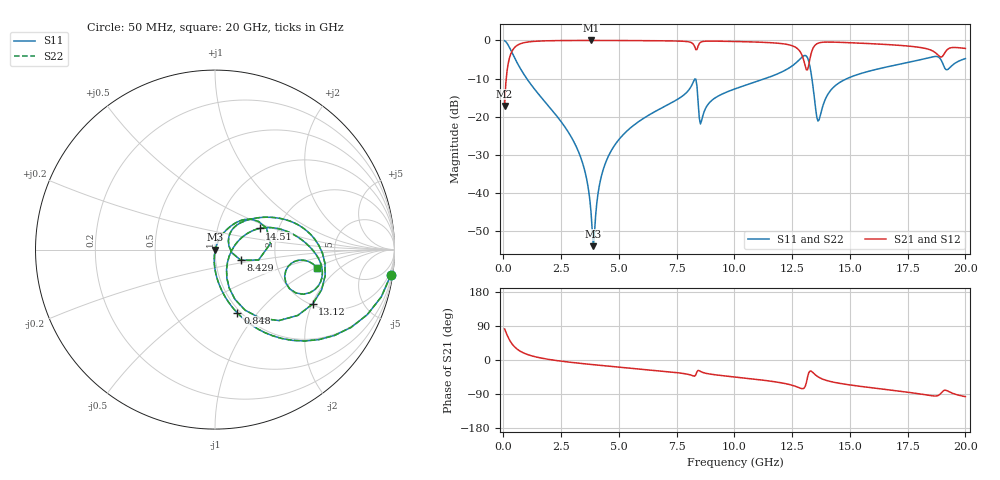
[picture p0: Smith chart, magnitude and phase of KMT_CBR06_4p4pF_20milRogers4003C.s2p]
! Data measured by Modelithics Inc. support@modelithics.com 813-866-6335
! KEMET CBR0603 4.4pF, Pad Width= 0.851mm, Pad Length= 0.64mm, Pad Gap= 0.62mm, 20mil Rogers 4003C substrate Data, January 2022
# hz S ma R 50
! 2 Port Network Data from SP1.SP block
! freq  magS11  angS11  magS21  angS21  magS12  angS12  magS22  angS22
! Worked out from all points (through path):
!   401 points, 50 MHz to 20 GHz, reference 50 ohm
!   highest |S21| = -0.02 dB at 3.791 GHz (marker M1); lowest = -17.2 dB at 50 MHz (marker M2)
!   group delay of S21, straight-line fit = 15.7 ps
!   lowest |S11| = -54.0 dB at 3.89 GHz (marker M3), VSWR 1.00, Z = 50.2 - j0.0729 ohm
!   |S11| at or under -10 dB: 1.007 GHz to 11.34 GHz (10.34 GHz wide, 167 % of centre); 13.35 GHz to 14.88 GHz (1.526 GHz wide, 10.8 % of centre)
!   |S22| runs from -54.0 to -0.1 dB; largest |S21 - S12| = 0
!   S11 on the Smith chart (normalised r, x): 50 MHz: 1, -14; 848 MHz: 0.97, -0.79; 8.429 GHz: 1.33, -0.16; 13.12 GHz: 2.04, -2.02; 14.51 GHz: 1.60, +0.41; 20 GHz: 3.40, -1.02
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5e7  0.9904 -8.1  0.138 81.9  0.138 81.9  0.9904 -8.1
2.99375e8  0.7657 -40.9  0.6424 49.0  0.6424 49.0  0.7657 -40.9
8.48e8  0.3742 -70.6  0.9263 19.3  0.9263 19.3  0.3742 -70.6
3.391625e9  0.02657 -95.3  0.9977 -9.3  0.9977 -9.3  0.02657 -95.3
3.641e9  0.01314 -92.5  0.9979 -10.8  0.9979 -10.8  0.01314 -92.5
3.790625e9  0.005649 -81.5  0.9979 -11.8  0.9979 -11.8  0.005649 -81.5
3.890375e9  0.002003 -21.2  0.9979 -12.4  0.9979 -12.4  0.002003 -21.2
4.2395e9  0.01654 68.4  0.9976 -14.4  0.9976 -14.4  0.01654 68.4
4.6385e9  0.03451 69.7  0.9971 -16.7  0.9971 -16.7  0.03451 69.7
6.73325e9  0.1245 60.1  0.9889 -28.5  0.9889 -28.5  0.1245 60.1
8.2295e9  0.2895 32.6  0.8842 -42.2  0.8842 -42.2  0.2895 32.6
8.429e9  0.1562 -22.5  0.844 -27.4  0.844 -27.4  0.1562 -22.5
8.578625e9  0.08853 32.5  0.9579 -31.6  0.9579 -31.6  0.08853 32.5
1.0025e10  0.2314 43.8  0.9673 -44.9  0.9673 -44.9  0.2314 43.8
1.251875e10  0.4672 18.5  0.8472 -67.0  0.8472 -67.0  0.4672 18.5
1.311725e10  0.6228 -29.2  0.4103 -59.1  0.4103 -59.1  0.6228 -29.2
1.336662e10  0.299 -68.1  0.7436 -31.5  0.7436 -31.5  0.299 -68.1
1.366588e10  0.09085 -6.6  0.9276 -46.0  0.9276 -46.0  0.09085 -6.6
1.451375e10  0.2752 25.4  0.9444 -61.2  0.9444 -61.2  0.2752 25.4
1.670825e10  0.4563 9.7  0.8787 -79.0  0.8787 -79.0  0.4563 9.7
1.895262e10  0.5505 -26.8  0.6041 -87.0  0.6041 -87.0  0.5505 -26.8
2e10  0.5767 -10.0  0.7841 -96.7  0.7841 -96.7  0.5767 -10.0
